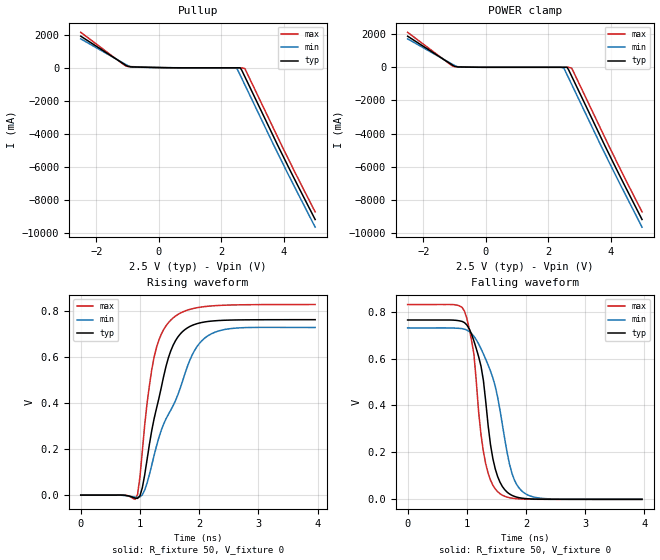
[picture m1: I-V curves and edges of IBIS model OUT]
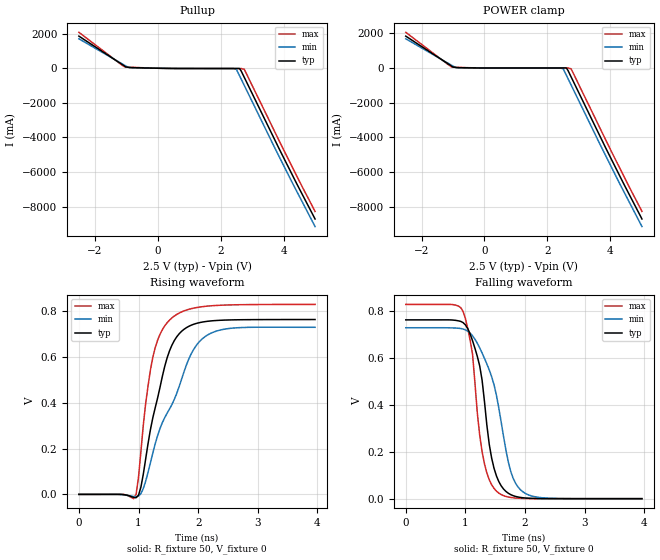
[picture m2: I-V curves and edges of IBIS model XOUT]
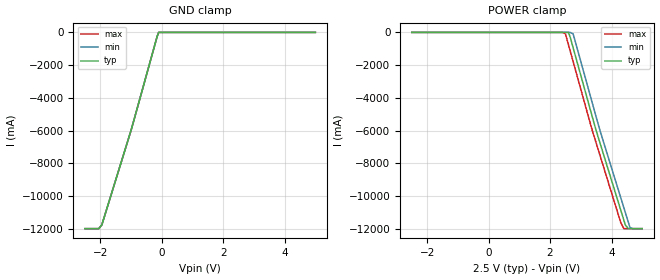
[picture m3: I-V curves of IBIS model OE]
|   IBIS File xg5032han_25v.ibs
[IBIS Ver]   3.2
[File name]   xg5032han_25v.ibs
[File Rev]   1.0
[Date]   April 5, 2013
[Source]
[Disclaimer]
Seiko Epson Corporation makes no warranty with respect to the information
contained herein.
[Copyright]
Copyright(C) 2013, Seiko Epson Corporation. All rights reserved.
|   Component XG5032HAN 2.5V
[Component]   xg5032han_25v
[Manufacturer]   Seiko Epson Corporation
[Package]
| variable   typ   min   max
R_pkg   0.07   NA   NA
L_pkg   0.9n   NA   NA
C_pkg   1p   NA   NA
[Pin]   signal_name   model_name   R_pin   L_pin   C_pin
1   OE   OE
2   GND   GND
3   GND   GND
4   OUT   OUT   0.05   0.5n   0.7p
5   XOUT   XOUT   0.09   1.2n   1.3p
6   VCC   POWER
[Diff Pin] inv_pin vdiff   tdelay_typ
4   5   0   0
| Models and submodels in the file (3): OUT (Open_source), XOUT (Open_source), OE (Input)
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[Model]   OUT
Model_type Open_source
Enable Active-High
Polarity Non-Inverting
Vref=0
Vmeas=0.375
Rref=50
Cref=0
C_comp   3.42p   3.33p   3.88p
[Temperature Range] 25   85   -40
[Voltage Range]   2.5   2.375   2.625
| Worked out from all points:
|   slope of the pullup table from 0 to 0.375 V, typ, clamps not added: 37.4 ohm
|   POWER clamp passes 1 mA (typ) near -0.18 V on its own axis
|   falling waveform, R_fixture 50, V_fixture 0: 20-80 % time 264ps typ, 385ps min, 219ps max; typ from 0.764 V to 0 V
|   rising waveform, R_fixture 50, V_fixture 0: 20-80 % time 379ps typ, 623ps min, 275ps max; typ from 0 V to 0.764 V
[Pullup]
-2.5V     1.9A       1.738A     2.133A
-1.05V    128.9mA    176.2mA    86.25mA
-900mV    42.69mA    43.36mA    57.46mA
-750mV    33.01mA    23.32mA    47.02mA
2.4V      -15.34mA   -14.87mA   -16.69mA
2.5V      -15.34mA   -60.94mA   -16.7mA
2.6V      -15.34mA   -452.5mA   -16.7mA
2.65V     -156.5mA   -650mA     -16.7mA
2.75V     -551.5mA   -1.045A    -62.1mA
3.7V      -4.304A    -4.796A    -3.811A
4.3V      -6.605A    -7.074A    -6.135A
5V        -9.201A    -9.663A    -8.74A
[POWER Clamp]
-2.5V     1.879A     1.718A     2.112A
-1.15V    236.4mA    271mA      194.2mA
-1V       60.22mA    110.5mA    44.66mA
-900mV    23.57mA    28.87mA    35.07mA
-750mV    15.78mA    9.161mA    27.12mA
2.4V      -141.5pA   -159.1pA   -132.5pA
2.5V      -149.5pA   -51.72mA   -140.5pA
2.6V      -157.5pA   -444.4mA   -148.5pA
2.75V     -543.1mA   -1.037A    -51.72mA
3.7V      -4.296A    -4.787A    -3.802A
4.3V      -6.597A    -7.066A    -6.126A
5V        -9.192A    -9.654A    -8.73A
[Falling Waveform]
R_fixture=50
V_fixture=0
V_fixture_min=0
V_fixture_max=0
0s        764.1mV    730.4mV    830.1mV
960ps     753.1mV    725mV      802.1mV
1.12ns    674.7mV    694.7mV    619.1mV
1.24ns    567mV      641.6mV    275mV
1.32ns    415.5mV    596.6mV    150.6mV
1.44ns    173.8mV    517.5mV    60.41mV
1.56ns    73.17mV    381.1mV    24.02mV
1.76ns    17.25mV    112.7mV    5.15mV
2ns       2.978mV    22.45mV    840.2uV
3.96ns    0V         0V         0V
[Rising Waveform]
R_fixture=50
V_fixture=0
V_fixture_min=0
V_fixture_max=0
0s        0V         939nV      0V
920ps     -13.42mV   -9.168mV   -18.46mV
960ps     -14.36mV   -9.902mV   3.299mV
1.04ns    31.66mV    1.311mV    189.7mV
1.12ns    153.9mV    51.98mV    399.1mV
1.24ns    333.6mV    173.5mV    601.9mV
1.56ns    652.3mV    389.1mV    771.5mV
1.92ns    742.9mV    628.6mV    813.7mV
2.2ns     757.6mV    701.5mV    823.6mV
3.96ns    764mV      730mV      830.1mV
[Ramp]
R_load=50
dV/dt_r   4.584E-1/3.776E-10   4.380E-1/6.231E-10   4.981E-1/2.727E-10
dV/dt_f   4.584E-1/2.615E-10   4.382E-1/3.836E-10   4.981E-1/2.165E-10
|[End   OUT
[Model]   XOUT
Model_type Open_source
Enable Active-High
Polarity Inverting
Vref=0
Vmeas=0.375
Rref=50
Cref=0
C_comp   3.42p   3.33p   3.88p
[Temperature Range] 25   85   -40
[Voltage Range]   2.5   2.375   2.625
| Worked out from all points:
|   slope of the pullup table from 0 to 0.375 V, typ, clamps not added: 37.4 ohm
|   POWER clamp passes 1 mA (typ) near -0.18 V on its own axis
|   falling waveform, R_fixture 50, V_fixture 0: 20-80 % time 263ps typ, 385ps min, 219ps max; typ from 0.764 V to 0 V
|   rising waveform, R_fixture 50, V_fixture 0: 20-80 % time 380ps typ, 624ps min, 276ps max; typ from 0 V to 0.764 V
[Pullup]
-2.5V     1.857A     1.703A     2.078A
-1.05V    126mA      172.7mA    85.19mA
-900mV    42.59mA    43.04mA    57.38mA
-750mV    32.98mA    23.3mA     46.96mA
400mV     -10.53mA   -8.097mA   -13.23mA
2.4V      -15.34mA   -14.87mA   -16.69mA
2.5V      -15.34mA   -57.65mA   -16.7mA
2.6V      -15.34mA   -426.7mA   -16.7mA
2.75V     -520.2mA   -986.2mA   -58.71mA
3.8V      -4.436A    -4.896A    -3.971A
4.55V     -7.143A    -7.58A     -6.704A
5V        -8.719A    -9.156A    -8.281A
[POWER Clamp]
-2.5V     1.837A     1.684A     2.058A
-1.15V    231.1mA    265.6mA    189.2mA
-1V       59.23mA    108.2mA    44.48mA
-900mV    23.52mA    28.64mA    35.04mA
-750mV    15.77mA    9.155mA    27.1mA
2.4V      -141.5pA   -159.1pA   -132.5pA
2.5V      -149.5pA   -49.23mA   -140.5pA
2.6V      -157.5pA   -419.6mA   -148.5pA
2.75V     -512.8mA   -979.1mA   -49.23mA
3.8V      -4.429A    -4.889A    -3.963A
4.55V     -7.135A    -7.573A    -6.695A
5V        -8.711A    -9.149A    -8.273A
[Falling Waveform]
R_fixture=50
V_fixture=0
V_fixture_min=0
V_fixture_max=0
0s        764.1mV    730.4mV    830.1mV
960ps     752.5mV    725.1mV    800.6mV
1.12ns    674.8mV    696mV      616.2mV
1.24ns    567.2mV    644.2mV    271mV
1.32ns    414.3mV    599.6mV    148.5mV
1.44ns    173.4mV    521.3mV    59.56mV
1.56ns    73.12mV    387.8mV    23.68mV
1.76ns    17.24mV    116.5mV    5.078mV
2ns       2.97mV     23.21mV    829.1uV
3.96ns    0V         0V         0V
[Rising Waveform]
R_fixture=50
V_fixture=0
V_fixture_min=0
V_fixture_max=0
0s        0V         1.688uV    0V
920ps     -13.54mV   -9.485mV   -18.77mV
960ps     -14.59mV   -10.01mV   1.277mV
1.04ns    31.76mV    3.669mV    187.2mV
1.12ns    155.2mV    57.79mV    397.7mV
1.24ns    335.1mV    181.1mV    599.5mV
1.56ns    652mV      392.7mV    771.1mV
1.88ns    738.8mV    612.4mV    811.1mV
2.2ns     757.5mV    702.4mV    823.6mV
3.96ns    764mV      730mV      830mV
[Ramp]
R_load=50
dV/dt_r   4.584E-1/3.787E-10   4.380E-1/6.237E-10   4.981E-1/2.738E-10
dV/dt_f   4.584E-1/2.607E-10   4.382E-1/3.830E-10   4.981E-1/2.154E-10
|[End   XOUT
[Model]   OE
Model_type Input
Vinh=1.75
Vinl=0.75
C_comp   3p   3p   3p
[Temperature Range] 25   85   -40
[Voltage Range]   2.5   2.375   2.625
[POWER Clamp Reference]2.5   2.375   2.625
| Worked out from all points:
|   GND clamp passes 1 mA (typ) near -0.10 V on its own axis
[GND Clamp]
-2.5V     -12A       -12A       -12A
-2.05V    -12A       -12A       -12A
-1.95V    -11.77A    -11.77A    -11.77A
-1V       -6A        -6A        -6A
-150mV    -254mA     -254mA     -254mA
-100mV    -25.23uA   -23.33uA   -29.37uA
5V        24.28uA    24.81uA    25.61uA
[POWER Clamp]
-2.5V     24.28uA    25.99uA    24.26uA
2.4V      -23.29uA   -20.27uA   -28.56uA
2.5V      -24.26uA   -21.21uA   -84.67mA
2.6V      -25.23uA   -22.15uA   -761.8mA
2.75V     -931.1mA   -84.67mA   -1.778A
3.35V     -4.994A    -4.148A    -5.84A
3.5V      -6A        -5.163A    -6.759A
4.3V      -10.86A    -10.1A     -11.62A
4.4V      -11.47A    -10.71A    -12A
4.45V     -11.77A    -11.01A    -12A
4.6V      -12A       -11.92A    -12A
5V        -12A       -12A       -12A
